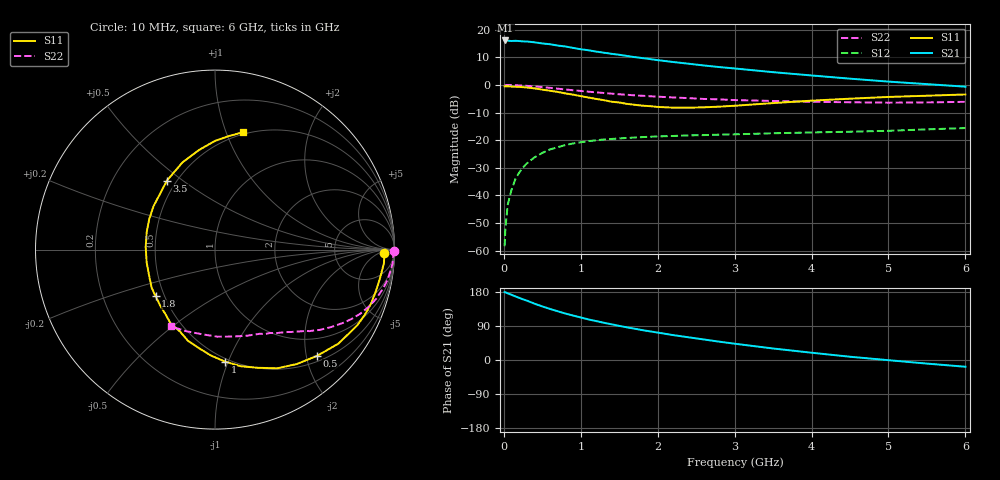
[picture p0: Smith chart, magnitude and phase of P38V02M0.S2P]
! SIEMENS Small Signal Semiconductors
! BFP181
! Si NPN RF Bipolar Junction Transistor in SOT143
! VCE = 8 V  IC = 2 mA
! Common Emitter S-Parameters:  March  1996
# GHz  S  MA  R  50
!  f  S11  S21  S12  S22
! GHz  MAG  ANG  MAG  ANG  MAG  ANG  MAG  ANG
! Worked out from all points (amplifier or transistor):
!   36 points, 10 MHz to 6 GHz, reference 50 ohm
!   highest |S21| = 16.1 dB at 20 MHz (marker M1)
!   |S21| within 3 dB of that: start of sweep to 962.7 MHz
!   unconditionally stable (mu >= 1): 2.575 GHz to end of sweep
!   at 250 MHz: K = 0.12, MSG = 22.8 dB, |S12| = -29.9 dB
!   at 1.4 GHz: K = 0.62, MSG = 15.4 dB, |S12| = -19.6 dB
!   at 6 GHz: K = 1.15, MAG = 5.1 dB, |S12| = -15.6 dB
!   lowest NFmin = 1.35 dB at 450 MHz
!   S11 on the Smith chart (normalised r, x): 10 MHz: 32, -9; 500 MHz: 0.61, -2.21; 1 GHz: 0.47, -0.97; 1.8 GHz: 0.45, -0.28; 3.5 GHz: 0.44, +0.44; 6 GHz: 0.48, +1.14
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0.01  0.9435 -1.0  6.351 179.1  0.0012 84.5  0.9962 -0.4
0.02  0.9431 -1.9  6.385 178.7  0.0025 91.1  0.991 -0.9
0.05  0.9444 -4.5  6.333 175.9  0.0067 90.0  0.9933 -2.3
0.1  0.9337 -9.5  6.24 172.0  0.0126 82.3  0.993 -4.5
0.15  0.9263 -14.3  6.293 167.9  0.0197 80.6  0.9852 -6.6
0.3  0.8974 -28.2  6.12 156.6  0.038 72.9  0.9612 -13.0
0.4  0.8645 -37.3  5.907 148.5  0.0489 67.3  0.9391 -17.0
0.5  0.8211 -46.1  5.632 141.4  0.0587 62.4  0.9129 -20.5
0.6  0.7839 -54.4  5.457 134.8  0.0678 57.5  0.8848 -23.8
0.7  0.7469 -62.3  5.16 128.6  0.0746 53.8  0.8548 -26.8
0.8  0.7008 -70.0  4.964 122.6  0.0812 50.0  0.8278 -29.3
1  0.6264 -84.9  4.425 112.2  0.0915 43.7  0.7776 -33.7
1.1  0.5907 -92.2  4.243 107.1  0.0959 40.8  0.7538 -35.7
1.3  0.5296 -106.6  3.833 98.3  0.1027 36.0  0.7137 -39.1
1.5  0.4804 -120.9  3.516 90.0  0.1073 32.6  0.677 -42.0
1.8  0.4208 -141.8  3.062 78.9  0.1134 28.5  0.6361 -46.0
2.2  0.3875 -169.4  2.599 65.7  0.1189 23.9  0.5918 -51.3
2.8  0.4039 155.1  2.105 48.4  0.1256 19.6  0.547 -59.2
3.5  0.4687 124.8  1.701 30.4  0.1331 16.1  0.5119 -69.6
4.5  0.563 98.9  1.298 8.6  0.142 11.9  0.4852 -88.5
5.5  0.637 83.1  1.033 -9.5  0.1565 10.2  0.4818 -109.1
6  0.6714 76.7  0.929 -17.8  0.1654 8.1  0.4938 -119.9
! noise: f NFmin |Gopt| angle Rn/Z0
0.45  1.35  0.6  17  0.4
0.9  1.45  0.5  36  0.4
1.8  1.8  0.31  80  0.37
